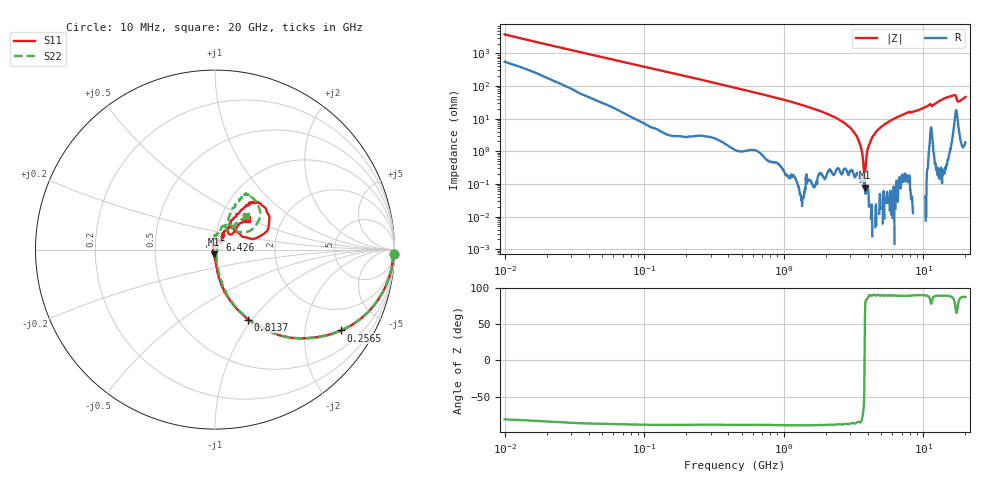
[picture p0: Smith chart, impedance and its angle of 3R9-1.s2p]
!Keysight Technologies,P5008B,MY61100088,A.16.20.02
!Date: Monday, May 27, 2024 15:21:29
!Correction: S11(C* 2-Port  )
!S21(C* 2-Port  )
!S12(C* 2-Port  )
!S22(C* 2-Port  )
!S2P File: Measurements: S11, S21, S12, S22:Log Frequency Sweep
# Hz S  dB  R 50
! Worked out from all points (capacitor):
!   1601 points, 10 MHz to 20 GHz, reference 50 ohm
!   read as one part in series: C = 4.26 pF near 10.39 MHz
!   lowest |Z| = 76.8 mohm at 3.793 GHz (marker M1)
!   series resonance near 3.789 GHz, so ESL is about 410 pH
!   S11 on the Smith chart (normalised r, x): 10 MHz: 6, -76; 256.5 MHz: 1.04, -3.10; 813.7 MHz: 1.00, -0.96; 6.426 GHz: 1.05, +0.11; 20 GHz: 1.34, +0.48
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1e7  -0.02 -1.5  -31.59 80.1  -31.61 80.1  -0.04 -1.5
3.555162e7  -0.08 -5.3  -20.59 81.6  -20.60 81.7  -0.08 -5.4
1.263918e8  -0.47 -17.8  -10.33 71.4  -10.35 71.4  -0.47 -17.8
2.565235e8  -1.57 -32.6  -5.42 56.3  -5.44 56.3  -1.57 -32.5
4.472136e8  -3.63 -48.4  -2.58 41.0  -2.59 41.0  -3.61 -48.2
8.137127e8  -7.30 -64.6  -0.93 25.1  -0.95 25.1  -7.29 -64.1
1.589917e9  -13.51 -78.9  -0.19 11.4  -0.21 11.4  -13.45 -77.3
2.70674e9  -20.87 -85.0  -0.03 3.3  -0.04 3.4  -20.81 -81.1
3.288784e9  -25.30 -90.1  -0.00 0.6  -0.01 0.6  -25.83 -79.2
3.792536e9  -31.12 -105.6  0.01 -1.4  -0.00 -1.4  -32.52 -64.2
4.072648e9  -35.11 -124.7  0.01 -2.4  -0.00 -2.4  -36.44 -42.2
4.436224e9  -38.49 -170.3  0.01 -3.7  0.00 -3.7  -38.94 4.5
5.652411e9  -28.95 80.5  0.01 -7.3  0.00 -7.3  -29.06 82.7
6.425969e9  -24.75 63.5  0.02 -9.3  0.00 -9.3  -25.19 87.7
7.697294e9  -20.99 58.6  -0.00 -12.7  -0.01 -12.7  -21.31 88.0
9.30816e9  -21.29 62.8  0.01 -16.6  -0.00 -16.6  -21.09 82.1
1.180378e10  -16.95 58.1  -0.12 -21.7  -0.14 -21.7  -16.95 66.7
1.335558e10  -11.81 56.7  -0.25 -27.0  -0.26 -26.9  -11.82 65.7
1.518335e10  -9.42 50.3  -0.52 -32.2  -0.53 -32.1  -9.36 61.4
1.661757e10  -8.88 37.5  -1.06 -35.6  -1.07 -35.6  -9.00 50.8
1.810106e10  -16.06 40.9  -0.35 -31.0  -0.36 -30.9  -15.91 47.1
2e10  -12.15 43.2  -0.38 -39.6  -0.39 -39.6  -11.90 46.8
